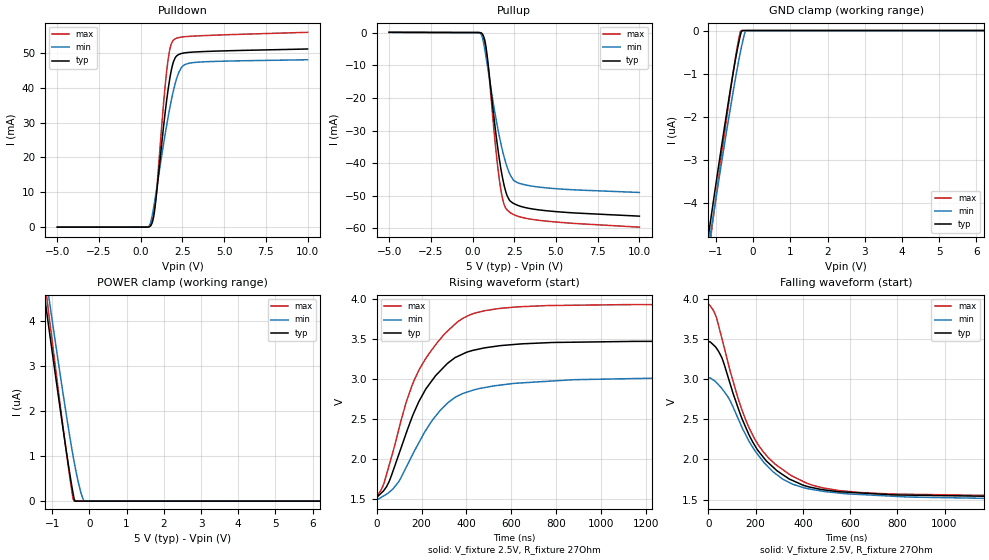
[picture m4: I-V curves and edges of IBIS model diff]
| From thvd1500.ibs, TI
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|   diff Model
[Model]   diff
Model_type   I/O
Polarity   Non-Inverting
Enable   Active-High
Vinl = 0.5
Vinh = 4.5
Vmeas = 2.5
Vref = 2.5
Cref = 2pF
Rref = 27
|   typ   min   max
C_comp   5.41561E-12   4.96197E-12   5.44074E-12
| Where Nom  PVT is Nominal Process, 5V, 27C
|   Fast PVT is Strong Process,  5.5V, -40C
|   Slow PVT is Weak Process,   4.5, 150C
[Voltage Range]   5   4.5   5.5
|Junction Temperature
[Temperature Range]   27   150   -40
[Pullup Reference]   5   4.5   5.5
[Pulldown Reference]   0   0   0
[Power Clamp Reference]   5   4.5   5.5
[GND Clamp Reference]   0   0   0
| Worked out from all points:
|   slope of the pulldown table from 0 to 0.75 V, typ, clamps not added: 317 ohm
|   slope of the pullup table from 0 to 0.75 V, typ, clamps not added: 269 ohm
|   falling waveform, V_fixture 2.5V, R_fixture 27Ohm: 20-80 % time 189ns typ, 197ns min, 191ns max; typ from 3.47 V to 1.54 V
|   rising waveform, V_fixture 2.5V, R_fixture 27Ohm: 20-80 % time 196ns typ, 208ns min, 204ns max; typ from 1.54 V to 3.47 V
[Pulldown]
|   Voltage   I(typ)   I(min)   I(max)
-5V       -17.2uA    -15.17uA   -19.09uA
370mV     -7.213uA   10.75uA    -10.13uA
580mV     305.6uA    1.058mA    450.5uA
760mV     2.55mA     5.172mA    3.554mA
895mV     7.231mA    9.156mA    7.709mA
1.36V     28.43mA    23.55mA    34.92mA
1.6V      37.98mA    30.42mA    46.5mA
1.795V    44.02mA    35.42mA    51.97mA
1.975V    47.58mA    39.41mA    53.67mA
2.44V     49.8mA     45.78mA    54.51mA
2.905V    50.13mA    47.01mA    54.71mA
10V       51.09mA    48mA       55.87mA
[GND Clamp]
|   Voltage   I(typ)   I(min)   I(max)
-5V       -28.56uA   -27.59uA   -31.74uA
-1.25V    -5.051uA   -5.31uA    -5.547uA
-1.04V    -3.805uA   -4.131uA   -4.149uA
-725mV    -1.993uA   -2.404uA   -2.114uA
-530mV    -948.4nA   -1.387uA   -937.2nA
-440mV    -514.3nA   -945.9nA   -452.4nA
-380mV    -254.8nA   -668nA     -167.4nA
-350mV    -137.8nA   -535.8nA   -43.89nA
-320mV    -30.77nA   -409.3nA   0A
-215mV    0A         -26.34nA   0A
-185mV    0A         0A         0A
10V       0A         0A         0A
[Pullup]
|   Voltage   I(typ)   I(min)   I(max)
-5V       79.83uA    77.21uA    73.21uA
355mV     11.12uA    -11.02uA   18.11uA
565mV     -298.8uA   -1.086mA   -422.9uA
760mV     -3.022mA   -6.008mA   -4.2mA
940mV     -10.03mA   -11.81mA   -10.54mA
1.375V    -30mA      -25.54mA   -34.79mA
1.66V     -40.54mA   -33.11mA   -46.94mA
1.9V      -46.96mA   -38.28mA   -52.76mA
2.2V      -51.26mA   -42.95mA   -54.94mA
2.485V    -52.41mA   -45.35mA   -55.8mA
3.535V    -53.97mA   -47.01mA   -57.18mA
10V       -56.22mA   -48.97mA   -59.6mA
[POWER Clamp]
|   Voltage   I(typ)   I(min)   I(max)
-5V       28.86uA    28.62uA    31.55uA
-1.25V    4.803uA    5.433uA    5.21uA
-1.055V   3.63uA     4.314uA    3.902uA
-605mV    1.021uA    1.829uA    990.5nA
-455mV    245.4nA    1.074uA    129.4nA
-440mV    176nA      1.004uA    54.01nA
-410mV    44.04nA    869.1nA    0A
-380mV    0A         737.5nA    0A
-230mV    0A         192.6nA    0A
-155mV    0A         17.2nA     0A
-125mV    0A         0A         0A
10V       0A         0A         0A
[Ramp]
R_load = 27
|   typ   min   max
dV/dt_r   1.16049/1.94374e-07   0.909014/2.06446e-07   1.4271/2.03491e-07
dV/dt_f   1.1605/1.87539e-07   0.909025/1.95457e-07   1.42712/1.91486e-07
[Falling Waveform]
V_fixture = 2.5V
V_fixture_min = 2.25V
V_fixture_max = 2.75V
R_fixture = 27Ohm
C_fixture = 0F
|   Time   V(typ)   V(min)   V(max)
0s        3.472V     3.019V     3.929V
32.23ns   3.394V     2.964V     3.782V
55.07ns   3.278V     2.891V     3.529V
127.4ns   2.627V     2.498V     2.743V
193.7ns   2.187V     2.123V     2.266V
256.2ns   1.952V     1.899V     2.015V
314.2ns   1.812V     1.756V     1.875V
413.9ns   1.668V     1.641V     1.708V
763.9ns   1.563V     1.545V     1.571V
2us       1.538V     1.503V     1.55V
[Rising Waveform]
V_fixture = 2.5V
V_fixture_min = 2.25V
V_fixture_max = 2.75V
R_fixture = 27Ohm
C_fixture = 0F
|   Time   V(typ)   V(min)   V(max)
0s        1.538V     1.503V     1.55V
25.76ns   1.591V     1.533V     1.649V
53.5ns    1.707V     1.581V     1.902V
133.2ns   2.336V     1.907V     2.723V
187.7ns   2.716V     2.203V     3.105V
284ns     3.103V     2.611V     3.5V
413.9ns   3.345V     2.846V     3.798V
553.9ns   3.417V     2.925V     3.882V
873.1ns   3.459V     2.99V      3.92V
2us       3.472V     3.018V     3.929V
